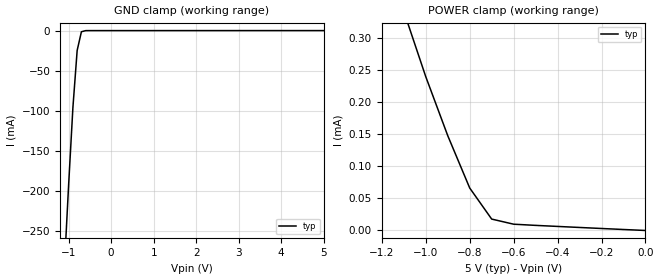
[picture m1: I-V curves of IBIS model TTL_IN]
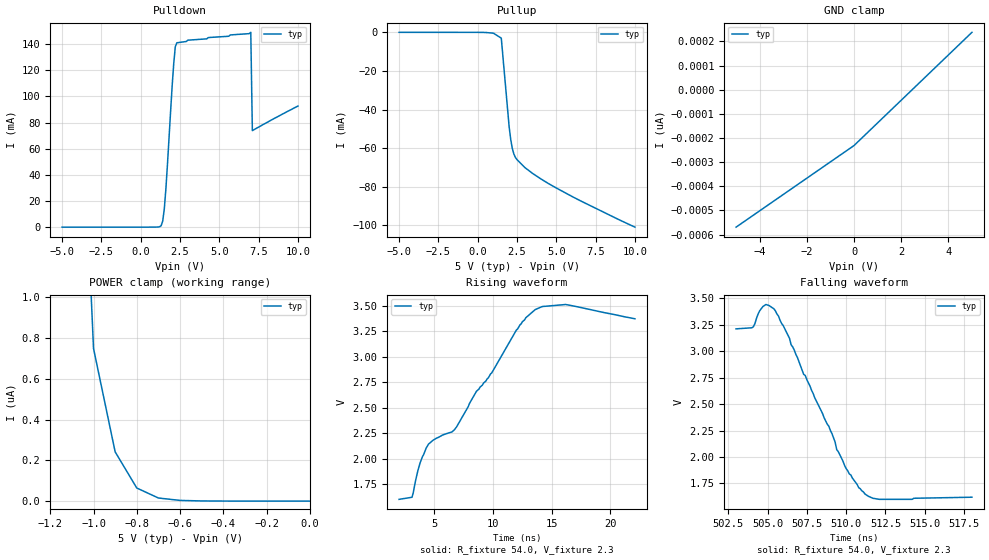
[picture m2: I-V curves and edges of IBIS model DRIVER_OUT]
|   Texas Instruments Incorporated
|   Data Transmissions Products
|   IBIS Model for SN75LBC172A
|   16N SOIC Package
[IBIS Ver]   3.2
[Comment char]   |_char
[File name]   lbc172an.ibs
[File Rev]   2.0
[Date]   16Jan01
[Source]   File originated at Texas Instruments Incorporated.
   Data Transmission Products Group. All data based on
   Bench Measurements.
[Notes]
[Disclaimer]
(C) Copyright Texas Instruments Incorporated 2001
   All rights reserved
  Texas Instruments Incorporated hereby grants the user of this IBIS
model a non-exclusive, nontransferable license to use this IBIS model
under the following terms.  Before using this IBIS model, the user
should read this license.  If the user does not accept these terms,
the IBIS model should be returned to Texas Instruments within 30 days.
  The user is granted this license only to use the IBIS model and
is not granted rights to sell, load, rent, lease or license the IBIS
model in whole or in part, or in modified form to anyone other than
user.  User may modify the IBIS model to suit its specific applications
but rights to derivative works and such modifications shall belong to
Texas Instruments.
  This IBIS model is provided on an "AS IS" basis and Texas Instruments
makes absolutely no warranty with respect to the information contained
herein.  TEXAS INSTRUMENTS DISCLAIMS AND CUSTOMER WAIVES ALL WARRANTIES,
EXPRESS OR IMPLIED, INCLUDING WARRANTIES OF MERCHANTABILITY OR FITNESS
FOR A PARTICULAR PURPOSE. The entire risk as to quality and performance
is with the Customer. ACCORDINGLY, IN NO EVENT SHALL THE COMPANY BE LIABLE
FOR ANY DAMAGES, WHETHER IN CONTRACT OR TORT,INCLUDING ANY LOST PROFITS
OR OTHER INCIDENTAL, CONSEQUENTIAL, EXEMPLARY, OR PUNITIVE DAMAGES ARISING
OUT OF THE USE OR APPLICATION OF THE IBIS model provided in this package.
Further, Texas Instruments reserves the right to discontinue or make changes
without notice to any product herein to improve reliability, function, or
design. Texas Instruments does not convey any license under patent rights
or any other intellectual property rights, including those of third parties.
Contact Texas Instruments at ATTN:DATA TRANSMISSIONS
[Copyright]   Copyright 2001, Texas Instruments, All Rights Reserved
[Component]   SN75LBC172AN
[Manufacturer]  Texas Instruments Incorporated
[Package]
|   typ   min   max
R_pkg   0.056   0.052   0.063
L_pkg   7.637nH   5.451nH   10.525nH
C_pkg   0.528pF   0.335pF   0.893pF
[Pin]   signal_name   model_name   R_pin   L_pin   C_pin
1   1A   TTL_IN   0.058   10.525n   0.892p
2   1Y   DRIVER_OUT   0.062   8.759n   0.535p
3   1Z   DRIVER_OUT   0.052   7.146n   0.387p
4   G   TTL_IN   0.053   5.451n   0.408p
5   2Z   DRIVER_OUT   0.053   5.513n   0.370p
6   2Y   DRIVER_OUT   0.053   6.304n   0.336p
7   2A   TTL_IN   0.057   7.830n   0.503p
8   GND   GND   0.056   9.581n   0.805p
9   3A   TTL_IN   0.058   9.603n   0.807p
10   3Y   DRIVER_OUT   0.062   7.864n   0.503p
11   3Z   DRIVER_OUT   0.052   6.295n   0.335p
12   /G   TTL_IN   0.053   5.499n   0.356p
13   4Z   DRIVER_OUT   0.053   5.452n   0.404p
14   4Y   DRIVER_OUT   0.053   7.156n   0.387p
15   4A   TTL_IN   0.063   8.740n   0.534p
16   VCC   POWER   0.056   10.478n   0.893p
[Diff_pin]   inv_pin   vdiff   tdelay_typ   tdelay_min   tdelay_max
| The 'xY' pin is Diff_pin and the 'xZ' pin is the inv_pin
2   3   NA   0 0 0
6   5   NA   0 0 0
10   11   NA   0 0 0
14   13   NA   0 0 0
| Models and submodels in the file (2): TTL_IN (Input), DRIVER_OUT (3-state)
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|   TTL Input Model
[Model]   TTL_IN
Model_type   Input
|Signals   G,/G,1A,2A,3A,4A
Vinh = 2.0
Vinl = 0.8
|   typ   min   max
C_comp   1.0pF   NA   NA
|   typ   min   max
[Temperature Range]   25.0   NA   NA
[Voltage range]   5.0V   4.75V   5.25V
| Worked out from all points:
|   GND clamp passes 1 mA (typ) near -0.67 V on its own axis
[GND_clamp]
|   Voltage   I(typ)   I(min)   I(max)
-5V       -4.21A     NA         NA
-2V       -1.22A     NA         NA
-1V       -192mA     NA         NA
-900mV    -96.1mA    NA         NA
-800mV    -24.8mA    NA         NA
-700mV    -1.47mA    NA         NA
-500mV    -28.2uA    NA         NA
5V        11.6pA     NA         NA
[Power_clamp]
| Note that the[POWER_clamp]voltage table is referenced to Vcc
| and is calculated using Vtable=Vcc - Vmeasured.
|   Voltage   I(typ)   I(min)   I(max)
-5V       4.42mA     NA         NA
-2V       1.26mA     NA         NA
-1V       240uA      NA         NA
-900mV    148uA      NA         NA
-800mV    66.3uA     NA         NA
-700mV    17.8uA     NA         NA
-600mV    9.8uA      NA         NA
0V        11.6pA     NA         NA
|   Driver Output Model
[Model]   DRIVER_OUT
Model_type   3-state
| Signals   1Y,1Z,2Y,2Z,3Y,3Z,4Y,4Z
Vmeas = 2.3V   |Reference voltage for timing measurements
Cref = 50pF   |Timing specification test load capacitance value
Rref = 54   |Note: 54 Ohm load; single ended configuration
|   typ   min   max
C_comp   1.0pF   NA   NA
|   typ   min   max
[Temperature Range]   25.0   NA   NA
[Voltage range]   5.0V   4.75V   5.25V
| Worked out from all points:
|   slope of the pulldown table from 0 to 0.75 V, typ, clamps not added: 18.8 kohm
|   slope of the pullup table from 0 to 0.75 V, typ, clamps not added: 3.08 kohm
|   rising waveform, R_fixture 54.0, V_fixture 2.3: 20-80 % time 7ns typ, NA min, NA max; typ from 1.6 V to 3.37 V
|   falling waveform, R_fixture 54.0, V_fixture 2.3: 20-80 % time 2.84ns typ, NA min, NA max; typ from 3.21 V to 1.62 V
[Pulldown]
|   Voltage   I(typ)   I(min)   I(max)
-5V       -560pA     NA         NA
1.3V      1.13mA     NA         NA
1.4V      4.65mA     NA         NA
1.5V      13.9mA     NA         NA
1.6V      29mA       NA         NA
2V        108mA      NA         NA
2.1V      125mA      NA         NA
2.2V      138mA      NA         NA
2.3V      141mA      NA         NA
7V        149mA      NA         NA
7.1V      73.8mA     NA         NA
10V       92.6mA     NA         NA
[Pullup]
|   Voltage   I(typ)   I(min)   I(max)
| Note that the[Pullup]voltage table is referenced to Vcc
| and is calculated using Vtable=Vcc - Vmeasured.
-5V       16.6uA     NA         NA
500mV     -60.3uA    NA         NA
1V        -426uA     NA         NA
1.5V      -3.01mA    NA         NA
2V        -49mA      NA         NA
2.1V      -55.5mA    NA         NA
2.2V      -60.2mA    NA         NA
2.4V      -64.9mA    NA         NA
3V        -70.1mA    NA         NA
4.5V      -78.4mA    NA         NA
6.5V      -87.2mA    NA         NA
10V       -101mA     NA         NA
| Output in High Impedance (off)
[GND_clamp]
|   Voltage   I(typ)   I(min)   I(max)
-5V       -569pA     NA         NA
0V        -231pA     NA         NA
5V        238pA      NA         NA
[POWER_clamp]
|   Voltage   I(typ)   I(min)   I(max)
| Note that the [POWER_clamp] voltage table is referenced to Vcc
| and is calculated using Vtable = Vcc - Vmeasured.
| Outputs in Tri-state.
-5V       16.6uA     NA         NA
-1.5V     12.7uA     NA         NA
-1V       749nA      NA         NA
-900mV    242nA      NA         NA
-800mV    64.6nA     NA         NA
-700mV    15.6nA     NA         NA
-600mV    3.78nA     NA         NA
0V        238pA      NA         NA
[Ramp]
|   typ   min   max
dV/dt_r   1.77v/7ns   NA   NA
dV/dt_f   1.60v/3.2ns   NA   NA
R_load = 54ohm  | Note: The measurement is single-ended with respect
|   to ground.
[Rising Waveform]
R_fixture = 54.0
V_fixture = 2.3
C_fixture = 0p
L_fixture = 0n
|   V(typ)   V(min)   V(max)
2ns       1.6V       NA         NA
3.1ns     1.62V      NA         NA
3.8ns     1.96V      NA         NA
4.5ns     2.14V      NA         NA
6.7ns     2.28V      NA         NA
9.9ns     2.84V      NA         NA
12ns      3.26V      NA         NA
13.6ns    3.46V      NA         NA
16.2ns    3.51V      NA         NA
22.1ns    3.37V      NA         NA
[Falling Waveform]
R_fixture = 54.0
V_fixture = 2.3
C_fixture = 0p
L_fixture = 0n
|   V(typ)   V(min)   V(max)
503ns     3.21V      NA         NA
504.1ns   3.23V      NA         NA
504.5ns   3.38V      NA         NA
504.9ns   3.44V      NA         NA
505.4ns   3.4V       NA         NA
508.9ns   2.29V      NA         NA
509.4ns   2.07V      NA         NA
511.2ns   1.65V      NA         NA
512.1ns   1.6V       NA         NA
518ns     1.62V      NA         NA
